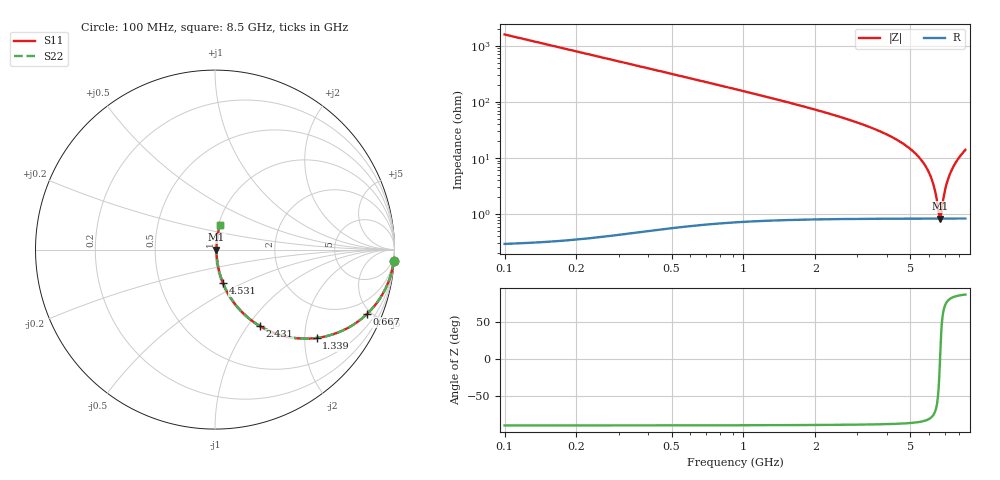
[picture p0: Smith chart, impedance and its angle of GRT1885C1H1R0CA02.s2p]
!Murata Part Number: GRT1885C1H1R0CA02
!These Parameters are Measured in Series Mode Connection
!Data Generated on Jun 19, 2026
!  o--ll--o
!Port1  Port2
!  o------o
!Operation Temp=25[degC], DC Bias Voltage=0[V]
!Freq. Start=100[MHz] Stop=9[GHz] 401[Steps]
# Hz S RI R 50
!Freq.(Hz) S11(Real) S11(Imag) S21(Real) S21(Imag) S12(Real) S12(Imag) S22(Real) S22(Imag)
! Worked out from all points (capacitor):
!   401 points, 100 MHz to 8.5 GHz, reference 50 ohm
!   read as one part in series: C = 1 pF near 142 MHz
!   lowest |Z| = 834 mohm at 6.652 GHz (marker M1)
!   series resonance near 6.655 GHz, so ESL is about 570 pH
!   S11 on the Smith chart (normalised r, x): 100 MHz: 1, -32; 667 MHz: 1.01, -4.72; 1.339 GHz: 1.02, -2.28; 2.431 GHz: 1.02, -1.14; 4.531 GHz: 1.02, -0.39; 8.5 GHz: 1.02, +0.28
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1e8  0.9961 -0.0626  0.00395 0.0626  0.00395 0.0626  0.9961 -0.0626
2.26e8  0.9801 -0.1394  0.0199 0.1394  0.0199 0.1394  0.9801 -0.1394
3.31e8  0.9581 -0.1998  0.0419 0.1998  0.0419 0.1998  0.9581 -0.1998
6.67e8  0.8472 -0.3584  0.1528 0.3584  0.1528 0.3584  0.8472 -0.3584
1.339e9  0.5656 -0.4923  0.4344 0.4923  0.4344 0.4923  0.5656 -0.4923
1.507e9  0.502 -0.4961  0.498 0.4961  0.498 0.4961  0.502 -0.4961
2.431e9  0.2496 -0.4257  0.7504 0.4257  0.7504 0.4257  0.2496 -0.4257
2.914e9  0.171 -0.3675  0.829 0.3675  0.829 0.3675  0.171 -0.3675
4.3e9  0.0542 -0.2085  0.9458 0.2085  0.9458 0.2085  0.0542 -0.2085
4.531e9  0.044 -0.1849  0.956 0.1849  0.956 0.1849  0.044 -0.1849
5.203e9  0.0232 -0.1208  0.9768 0.1208  0.9768 0.1208  0.0232 -0.1208
5.707e9  0.0142 -0.0765  0.9858 0.0765  0.9858 0.0765  0.0142 -0.0765
6.001e9  0.011 -0.0519  0.989 0.0519  0.989 0.0519  0.011 -0.0519
6.232e9  0.00937 -0.0332  0.9906 0.0332  0.9906 0.0332  0.00937 -0.0332
6.379e9  0.00873 -0.0215  0.9913 0.0215  0.9913 0.0215  0.00873 -0.0215
6.589e9  0.00829 -0.00511  0.9917 0.00511  0.9917 0.00511  0.00829 -0.00511
6.652e9  0.00827 -0.000242  0.9917 0.000242  0.9917 0.000242  0.00827 -0.000242
6.715e9  0.00829 0.0046  0.9917 -0.0046  0.9917 -0.0046  0.00829 0.0046
6.925e9  0.0087 0.0205  0.9913 -0.0205  0.9913 -0.0205  0.0087 0.0205
7.114e9  0.00949 0.0347  0.9905 -0.0347  0.9905 -0.0347  0.00949 0.0347
7.66e9  0.0139 0.0746  0.9861 -0.0746  0.9861 -0.0746  0.0139 0.0746
8.5e9  0.0269 0.1346  0.9731 -0.1346  0.9731 -0.1346  0.0269 0.1346
